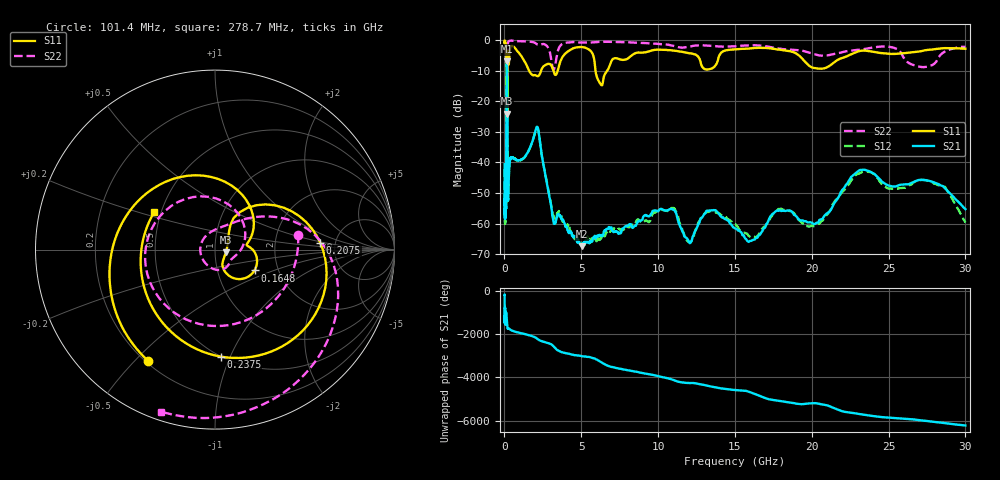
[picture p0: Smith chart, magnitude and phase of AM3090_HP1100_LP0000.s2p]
! Date/Time: Thu, Feb 28, 2019 2:06 PM
! Network Analyzer: Agilent Technologies E8364B Rev: A.07.50.67
! Sweep from 0.010 to 30.000 GHz, 1601 Points, Sweep Type: LOG
! Power Supply: 5.023 V, 0.002 A
# Hz S DB R 50
!freq MagS11 AngS11 MagS21 AngS21 MagS12 AngS12 MagS22 AngS22
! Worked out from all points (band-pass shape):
!   1601 points, 10 MHz to 30 GHz, reference 50 ohm
!   highest |S21| = -7.01 dB at 156.8 MHz (marker M1); lowest = -67.3 dB at 5.027 GHz (marker M2)
!   |S21| within 3 dB of the highest: 139.5 MHz to 179.1 MHz (39.62 MHz wide, 24.9 % of centre)
!   lowest |S11| = -24.1 dB at 184.9 MHz (marker M3), VSWR 1.13, Z = 56.4 - j1.75 ohm
!   |S11| at or under -10 dB: 1.604 GHz to 2.382 GHz (777.2 MHz wide, 39 % of centre); 3.185 GHz to 3.466 GHz (280.6 MHz wide, 8.44 % of centre); 5.926 GHz to 6.694 GHz (768.3 MHz wide, 12.2 % of centre)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
!   |S22| runs from -21.7 to -0.1 dB; largest |S21 - S12| = 0.014
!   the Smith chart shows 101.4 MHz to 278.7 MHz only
!   S11 on the Smith chart (normalised r, x): 101.4 MHz: 0.21, -0.55; 164.8 MHz: 1.51, -0.37; 207.5 MHz: 3.79, +0.44; 237.5 MHz: 0.50, -0.92; 278.7 MHz: 0.46, +0.23
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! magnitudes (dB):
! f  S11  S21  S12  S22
! 10 MHz  -0.3  -40.6  -42.5  -0.5
! 38.04 MHz  -0.4  -56.2  -59.5  -1.1
! 48.61 MHz  -0.6  -49.0  -49.0  -1.3
! 101.4 MHz  -2.8  -55.2  -52.8  -6.5
! 144.7 MHz  -14.6  -8.0  -8.0  -18.6
! 156.8 MHz  -13.0  -7.0  -7.0  -18.6
! 164.8 MHz  -12.1  -7.3  -7.3  -20.2
! 184.9 MHz  -24.1  -13.6  -13.6  -13.5
! 207.5 MHz  -4.6  -47.8  -48.4  -2.4
! 237.5 MHz  -4.5  -51.9  -51.0  -0.8
! 278.7 MHz  -8.0  -45.3  -45.6  -0.4
! 550.5 MHz  -2.1  -38.4  -38.5  -0.2
! 2.084 GHz  -11.7  -28.6  -28.6  -1.2
! 3.204 GHz  -10.3  -59.7  -57.8  -9.6
! 5.027 GHz  -2.3  -67.3  -66.5  -0.8
! 6.202 GHz  -14.0  -63.7  -65.2  -0.6
! 7.926 GHz  -6.3  -60.7  -61.4  -0.7
! 13.54 GHz  -9.2  -55.6  -56.0  -1.9
! 16.13 GHz  -2.7  -65.4  -64.3  -1.7
! 20.31 GHz  -9.2  -59.7  -60.5  -4.8
! 23.48 GHz  -3.5  -42.4  -43.0  -2.9
! 30 GHz  -2.8  -55.2  -59.6  -2.2
